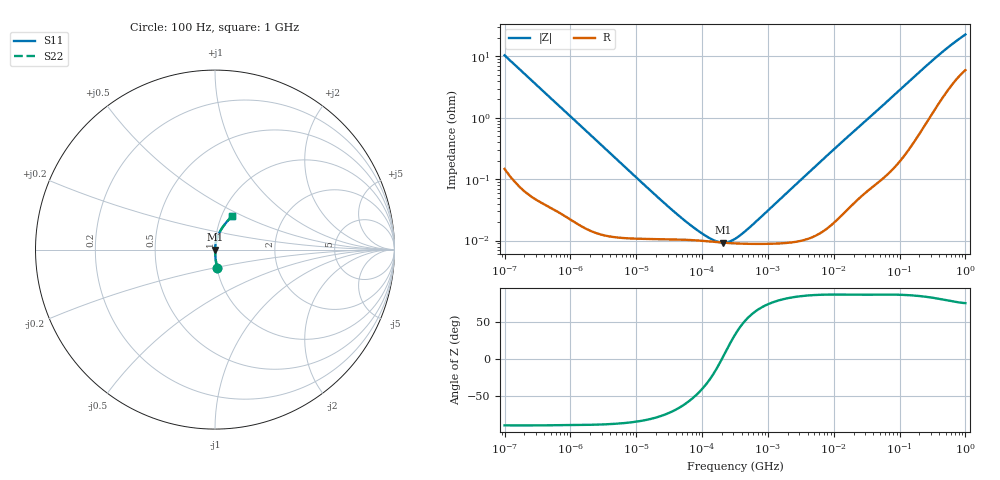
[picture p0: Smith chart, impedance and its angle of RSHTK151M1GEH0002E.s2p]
! RSHTK151M1GEH0002E  S-PARAMETER MODEL  (General Type)
! Model Generated by ELNA Corporation (http://www.ty-top.com)
! Version 1.0
! ELNA Control No. 201216
! Copyright (c) 2020 ELNA CO.,LTD. All Rights Reserved.
! Products Name : CONDUCTIVE POLYMER HYBRID ALUMINUM ELECTROLYTIC CAPACITORS
! Characteristics :
!  Capacitance  :  150uF  ,  Rated voltage  :  35V
!  Operating Temp. Range  :  -55 to +125 degC  ,  Endurance  :  4000hr at 125 degC
!  Dimension D  :  8mm  ,  Dimension L  :  10mm
! Frequency Range : 100Hz - 1GHz
! External Node Assignments :
!  1  o---| |---o  2
# MHz S RI R 50
!Freq[MHz].  S11 Real  S11 Imag  S21 Real  S21 Imag  S12 Real  S12 Imag  S22 Real  S22 Imag
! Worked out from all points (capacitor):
!   401 points, 100 Hz to 1 GHz, reference 50 ohm
!   read as one part in series: C = 153 uF near 108 Hz
!   lowest |Z| = 9.26 mohm at 211.3 kHz (marker M1)
!   series resonance near 200.4 kHz, so ESL is about 4.1 nH
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0.0001  0.0122 -0.1028  0.9878 0.1028  0.9878 0.1028  0.0122 -0.1028
0.000113  0.00966 -0.0914  0.9903 0.0914  0.9903 0.0914  0.00966 -0.0914
0.000183  0.00392 -0.0567  0.9961 0.0567  0.9961 0.0567  0.00392 -0.0567
0.000309  0.0016 -0.0337  0.9984 0.0337  0.9984 0.0337  0.0016 -0.0337
0.001488  0.00022 -0.00711  0.9998 0.00711  0.9998 0.00711  0.00022 -0.00711
0.022131  0.000106 -0.000477  0.9999 0.000477  0.9999 0.000477  0.000106 -0.000477
0.053703  0.000103 -0.000188  0.9999 0.000188  0.9999 0.000188  0.000103 -0.000188
0.106537  9.85e-05 -7.61e-05  0.9999 7.61e-05  0.9999 7.61e-05  9.85e-05 -7.61e-05
0.135675  9.63e-05 -4.59e-05  0.9999 4.59e-05  0.9999 4.59e-05  9.63e-05 -4.59e-05
0.153109  9.52e-05 -3.16e-05  0.9999 3.16e-05  0.9999 3.16e-05  9.52e-05 -3.16e-05
0.211349  9.24e-05 6.31e-06  0.9999 -6.31e-06  0.9999 -6.31e-06  9.24e-05 6.31e-06
0.269153  9.08e-05 3.59e-05  0.9999 -3.59e-05  0.9999 -3.59e-05  9.08e-05 3.59e-05
0.316228  8.99e-05 5.71e-05  0.9999 -5.71e-05  0.9999 -5.71e-05  8.99e-05 5.71e-05
0.402717  8.9e-05 9.21e-05  0.9999 -9.21e-05  0.9999 -9.21e-05  8.9e-05 9.21e-05
0.555904  8.83e-05 0.000148  0.9999 -0.000148  0.9999 -0.000148  8.83e-05 0.000148
4.704354  0.000115 0.00144  0.9999 -0.00144  0.9999 -0.00144  0.000115 0.00144
69.9842  0.00167 0.0198  0.9983 -0.0198  0.9983 -0.0198  0.00167 0.0198
176.8072  0.00682 0.0486  0.9932 -0.0486  0.9932 -0.0486  0.00682 0.0486
380.1894  0.0255 0.0968  0.9745 -0.0968  0.9745 -0.0968  0.0255 0.0968
668.3439  0.0594 0.1471  0.9406 -0.1471  0.9406 -0.1471  0.0594 0.1471
922.5714  0.0875 0.1793  0.9125 -0.1793  0.9125 -0.1793  0.0875 0.1793
1000  0.0953 0.1878  0.9047 -0.1878  0.9047 -0.1878  0.0953 0.1878
